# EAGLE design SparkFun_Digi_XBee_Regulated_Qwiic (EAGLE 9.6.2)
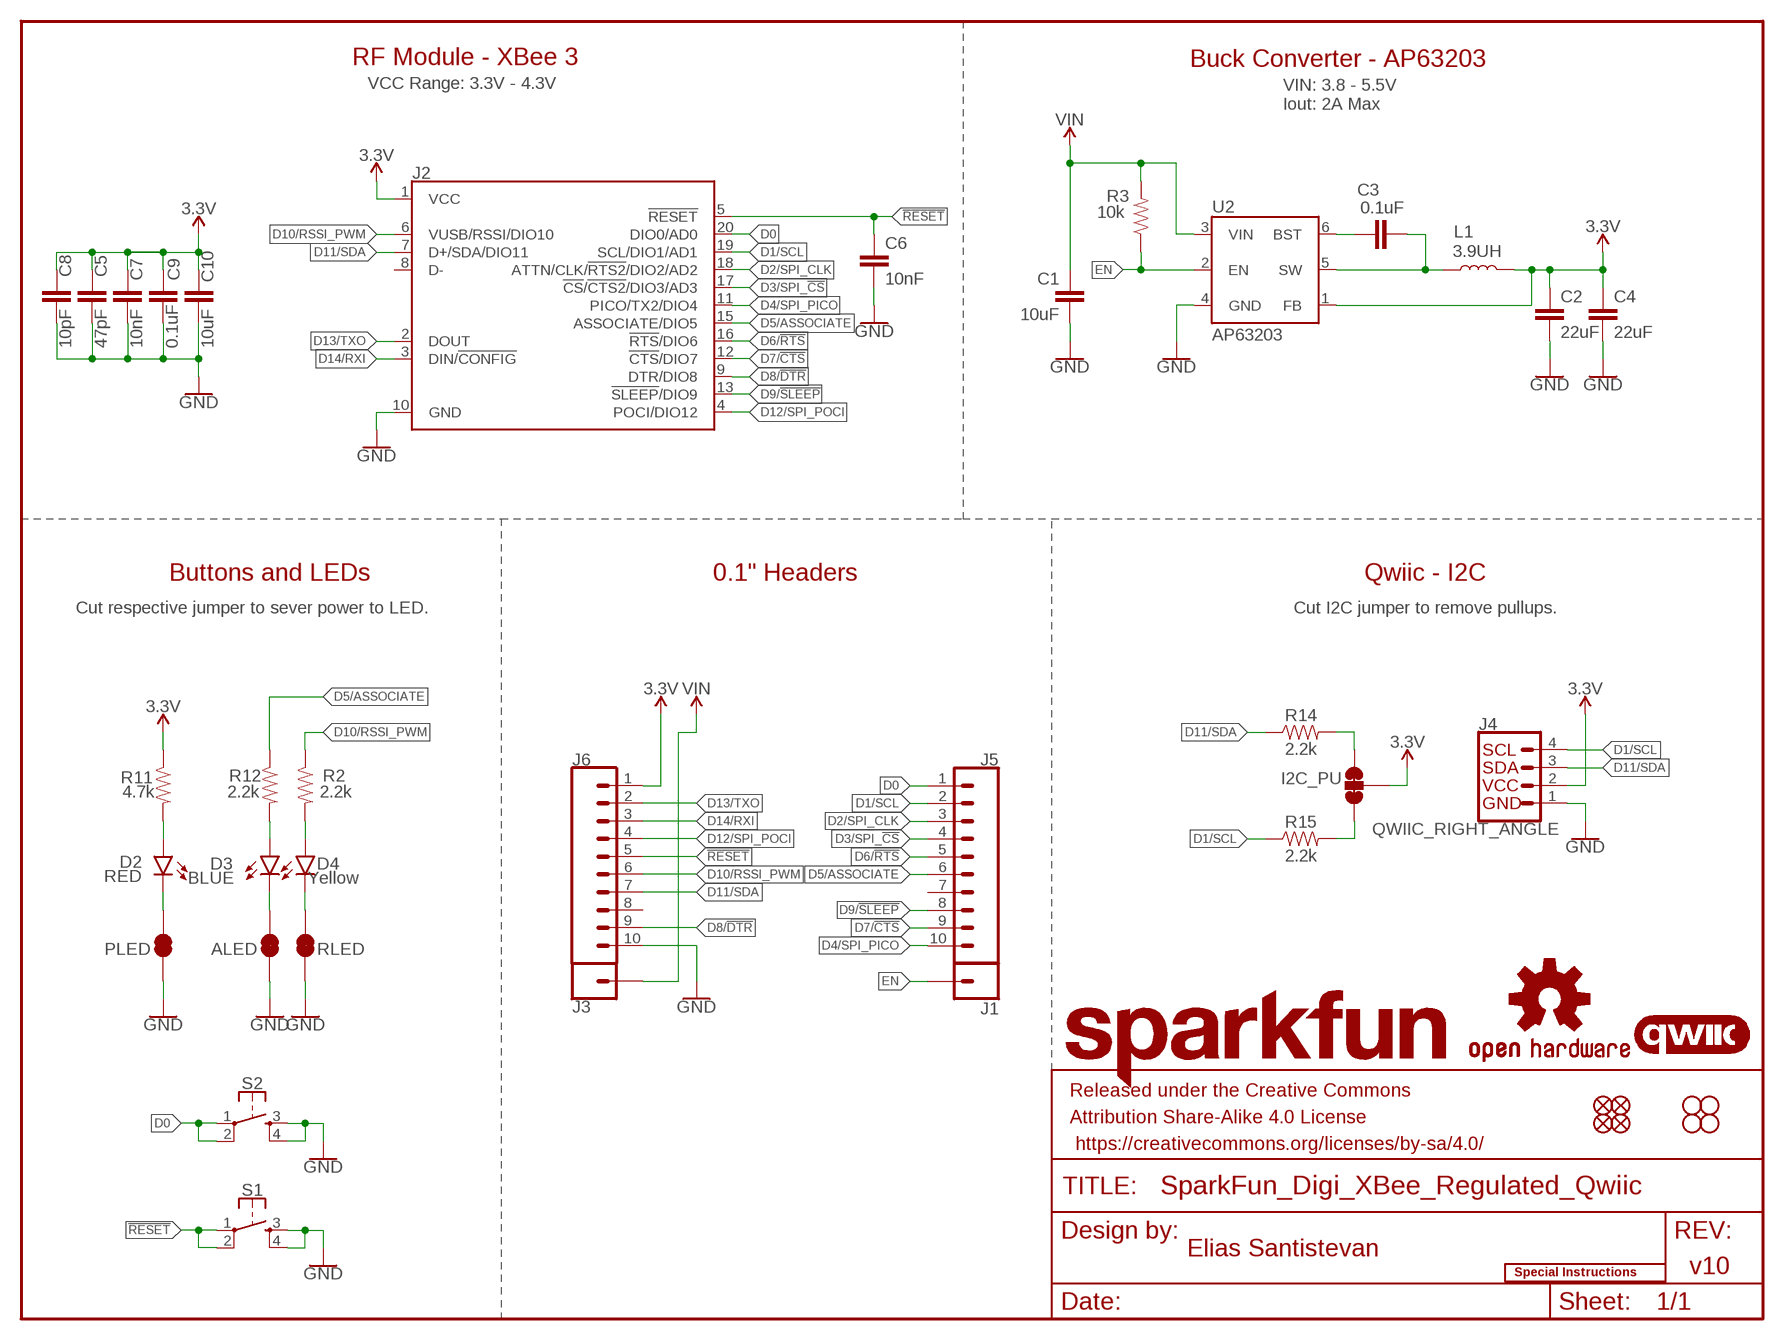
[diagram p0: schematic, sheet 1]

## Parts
ALED  JUMPER-SMT_2_NC_TRACE_SILK  [SMT-JUMPER_2_NC_TRACE_SILK]
C1  10uF  10UF-1210-50V-20%  [1210]
C2  22uF  22UF-0603-6.3V-20%  [0603]
C3  0.1uF  0.1UF-0603-25V-5%  [0603]
C4  22uF  22UF-0603-6.3V-20%  [0603]
C5  47pF  47PF-0603-50V-5%  [0603]
C6  10nF  10NF-0603-50V-10%  [0603]
C7  10nF  10NF-0603-50V-10%  [0603]
C8  10pF  10PF-0603-50V-5%  [0603]
C9  0.1uF  0.1UF-0603-25V-(+80/-20%)  [0603]
C10  10uF  10UF-0603-6.3V-20%  [0603]
D2  RED  LED-RED_0603-KB  [LED-0603]
D3  BLUE  LED-BLUE0603  [LED-0603]
D4  Yellow  LED-YELLOW0603  [LED-0603]
FD1  FIDUCIAL1X2  [FIDUCIAL-1X2]
FD2  FIDUCIAL1X2  [FIDUCIAL-1X2]
FD3  FIDUCIAL1X2  [FIDUCIAL-1X2]
FD4  FIDUCIAL1X2  [FIDUCIAL-1X2]
FRAME2  FRAME-LETTER  [CREATIVE_COMMONS]
H1  STAND-OFFTIGHT  [STAND-OFF-TIGHT]
H2  STAND-OFFTIGHT  [STAND-OFF-TIGHT]
H3  STAND-OFFTIGHT  [STAND-OFF-TIGHT]
H4  STAND-OFFTIGHT  [STAND-OFF-TIGHT]
I2C_PU  JUMPER-SMT_3_2-NC_TRACE_SILK  [SMT-JUMPER_3_2-NC_TRACE_SILK]
J1  CONN_01PTH_NO_SILK_STAND  [1X01_NO_SILK_STAND]
J2  XBEE_UPDATEXBEE_SMD  [XBEE3-SMD]
J3  CONN_01PTH_NO_SILK_STAND  [1X01_NO_SILK_STAND]
J4  QWIIC_RIGHT_ANGLE  QWIIC_CONNECTORJS-1MM  [JST04_1MM_RA]
J5  CONN_10NO_SILK_PTH_FEMALE  [1X10_NO_SILK]
J6  CONN_10NO_SILK_PTH_FEMALE  [1X10_NO_SILK]
L1  3.9UH  [INDUCTOR_3.9UH]
LOGO1  SPECIAL_INSTRUCTIONS-ORDERING  [ORDERING_INSTRUCTIONS]
LOGO2  OSHW-LOGOS  [OSHW-LOGO-S]
LOGO3  QWIIC_LOGO_4MM  [QWIIC_4MM]
LOGO4  SFE_LOGO_NAMEBLANK  [BLANK]
PLED  JUMPER-SMT_2_NC_TRACE_SILK  [SMT-JUMPER_2_NC_TRACE_SILK]
R2  2.2k  2.2KOHM-0603-1/10W-1%  [0603]
R3  10k  10KOHM-0603-1/10W-1%  [0603]
R11  4.7k  4.7KOHM-0603-1/10W-1%  [0603]
R12  2.2k  2.2KOHM-0603-1/10W-1%  [0603]
R14  2.2k  2.2KOHM-0603-1/10W-1%  [0603]
R15  2.2k  2.2KOHM-0603-1/10W-1%  [0603]
RLED  JUMPER-SMT_2_NC_TRACE_SILK  [SMT-JUMPER_2_NC_TRACE_SILK]
S1  MOMENTARY-SWITCH-SPST-2-SMD-5.2MM-TALL  [TACTILE_SWITCH_SMD_5.2MM]
S2  MOMENTARY-SWITCH-SPST-2-SMD-5.2MM-TALL  [TACTILE_SWITCH_SMD_5.2MM]
U2  AP63203  [SOT23-6]

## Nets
3.3V: C2.1 C4.1 C5.1 C7.1 C8.1 C9.1 C10.1 I2C_PU.2 J2.1(VCC) J4.2 J6.1 L1.P$2 R11.1 U2.1(FB)
!RESET!: C6.1 J2.5(!RESET!) J6.5 S1.1 S1.2
D0: J2.20(DIO0/AD0) J5.1 S2.1 S2.2
D1/SCL: J2.19(SCL/DIO1/AD1) J4.4 J5.2 R15.1
D2/SPI_CLK: J2.18(ATTN/CLK/!RTS2!/DIO2/AD2) J5.3
D3/SPI_!CS!: J2.17(!CS!/!CTS2!/DIO3/AD3) J5.4
D4/SPI_PICO: J2.11(PICO/TX2/DIO4) J5.10
D5/ASSOCIATE: J2.15(ASSOCIATE/DIO5) J5.6 R12.1
D6/!RTS!: J2.16(!RTS!/DIO6) J5.5
D7/!CTS!: J2.12(!CTS!/DIO7) J5.9
D8/!DTR!: J2.9(DTR/DIO8) J6.9
D9/!SLEEP!: J2.13(!SLEEP!/DIO9) J5.8
D10/RSSI_PWM: J2.6(VUSB/RSSI/DIO10) J6.6 R2.1
D11/SDA: J2.7(D+/SDA/DIO11) J4.3 J6.7 R14.1
D12/SPI_POCI: J2.4(POCI/DIO12) J6.4
D13/TXO: J2.2(DOUT) J6.2
D14/RXI: J2.3(DIN/!CONFIG!) J6.3
EN: J1.1 R3.1 U2.2(EN)
GND: ALED.1 C1.2 C2.2 C4.2 C5.2 C6.2 C7.2 C8.2 C9.2 C10.2 J2.10(GND) J4.1 J6.10 PLED.1 RLED.1 S1.3 S1.4 S2.3 S2.4 U2.4(GND)
N$1: C3.1 U2.6(BST)
N$2: D4.A R2.2
N$3: D4.C RLED.2
N$7: D2.A R11.2
N$8: C3.2 L1.P$1 U2.5(SW)
N$11: I2C_PU.3 R14.2
N$12: D3.A R12.2
N$13: I2C_PU.1 R15.2
N$21: ALED.2 D3.C
N$23: D2.C PLED.2
VIN: C1.1 J3.1 R3.2 U2.3(VIN)
Unconnected: J2.8(D-) J5.7 J6.8

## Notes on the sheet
- RF Module - XBee 3 | Buck Converter - AP63203
- VCC Range: 3.3V - 4.3V
- VIN: 3.8 - 5.5V
  Iout: 2A Max
- Buttons and LEDs | 0.1" Headers | Qwiic - I2C
- Cut respective jumper to sever power to LED. | Cut I2C jumper to remove pullups.
- Elias Santistevan
- v10

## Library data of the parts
ALED PLED RLED = SparkFun-Jumpers:JUMPER-SMT_2_NC_TRACE: Normally closed trace jumper
C1 = SparkFun-Capacitors:10UF: 10.0µF ceramic capacitors; PROD_ID: CAP-09824
C2 C4 = SparkFun-Capacitors:22UF: 22µF ceramic capacitors; PROD_ID: CAP-14464
C3 = SparkFun-Capacitors:0.1UF: 0.1µF ceramic capacitors; PROD_ID: CAP-08604
C5 = SparkFun-Capacitors:47PF: 47pF ceramic capacitors; PROD_ID: CAP-08913
C6 C7 = SparkFun-Capacitors:10NF: 0.01uF/10nF/10,000pF ceramic capacitors; PROD_ID: CAP-00867
C8 = SparkFun-Capacitors:10PF: 10pF ceramic capacitors; PROD_ID: CAP-11812
C9 = SparkFun-Capacitors:0.1UF: 0.1µF ceramic capacitors; PROD_ID: CAP-00810
C10 = SparkFun-Capacitors:10UF: 10.0µF ceramic capacitors; PROD_ID: CAP-11015
D2 = SparkFun-LED:LED-RED: Red SMD LED; PROD_ID: DIO-17976
D3 = SparkFun-LED:LED-BLUE: Blue SMD LED; PROD_ID: DIO-08575
D4 = SparkFun-LED:LED-YELLOW: Yellow SMD LED; PROD_ID: DIO-09003
FD1-FD4 = SparkFun-Aesthetics:FIDUCIAL: Fiducial Alignment Points
FRAME2 = SparkFun-Aesthetics:FRAME-LETTER: Schematic Frame - Letter
H1-H4 = SparkFun-Hardware:STAND-OFF: Stand Off
I2C_PU = SparkFun-Jumpers:JUMPER-SMT_3_2-NC_TRACE: Normally closed trace jumper (2 of 2 connections) This jumper has a trace between all three pads so they are normally closed (NC). Use a razor knife to open the connection(s). For best results follow the IPC guidelines for cutting traces: Cutout at least 0.063 mm (0.005 in). Remove all loose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
J1 J3 = SparkFun-Connectors:CONN_01: Single connection point. Often used as Generic Header-pin footprint for 0.1 inch spaced/style header connections
J2 = xbee_smart_modem:XBEE_UPDATE: XBee 3 Cat 1 Smart Modem
J4 = SparkFun-Connectors:QWIIC_CONNECTOR: SparkFun I2C Standard Qwiic Connector An SMD 1mm pitch JST connector makes it easy and quick (get it? Qwiic?) to connect I2C devices to each other. The Qwiic system enables fast and solderless connection between popular platforms and various sensors and actuators. We carry 200mm, 100mm, 50mm, and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; PROD_ID: CONN-13694
J5 J6 = SparkFun-Connectors:CONN_10: Multi connection point. Often used as Generic Header-pin footprint for 0.1 inch spaced/style header connections On any of the 0.1 inch spaced packages, you can populate with these: Break Away Headers - Straight (PRT-00116) Break Away Male Headers - Right Angle (PRT-00553) Female Headers (PRT-00115)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
L1 = SparkFun-Coils:3.9UH: Würth's Electronik 3.9uH Inductor; PROD_ID: NDUC-18014
LOGO1 = SparkFun-Aesthetics:SPECIAL_INSTRUCTIONS: Special Ordering/Production Instructions Alert
LOGO2 = SparkFun-Aesthetics:OSHW-LOGO: Open-Source Hardware (OSHW) Logo
LOGO3 = SparkFun-Aesthetics:QWIIC_LOGO: Qwiic Logos for placement on schematic and PCB. The 5.5mm silk logo is best for placing next to Qwiic connector.
LOGO4 = SparkFun-Aesthetics:SFE_LOGO_NAME: SparkFun Font Logo
R2 R12 R14 R15 = SparkFun-Resistors:2.2KOHM: 2.2kΩ resistor; PROD_ID: RES-08272
R3 = SparkFun-Resistors:10KOHM: 10kΩ resistor; PROD_ID: RES-00824
R11 = SparkFun-Resistors:4.7KOHM: 4.7kΩ resistor; PROD_ID: RES-07857
S1 S2 = SparkFun-Switches:MOMENTARY-SWITCH-SPST-2: Momentary Switch (Pushbutton) - SPST - Two Circuits Normally-open (NO) SPST momentary switches (buttons, pushbuttons). Schematic symbol includes two switch circuits. Variants SMD-4.6MMX2.8MM - 4.60mm x 2.80mm Tactile Momentary Button Switch - Used on SparkFun Pro Micro - RP2040 SMD-5.2MM - Mini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; PROD_ID: SWCH-14139
U2 = SparkFun-IC-Power:AP63203: Diodes Inc. AP63203 3.8V-32V input 3.3V Buck The AP63200/AP63201/AP63203/AP63205 is a 2A, synchronous buck converter with a wide input voltage range of 3.8V to 32V and fully integrates a 125mΩ high-side power MOSFET and a 68mΩ lowside power MOSFET to provide high-efficiency step-down DC/DC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; PROD_ID: VREG-15244

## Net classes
1 POWER: width 0.559 mm, drill 0.305 mm
2 Diff pairs: width 0.203 mm, drill 0.305 mm, clearance 0.152 mm

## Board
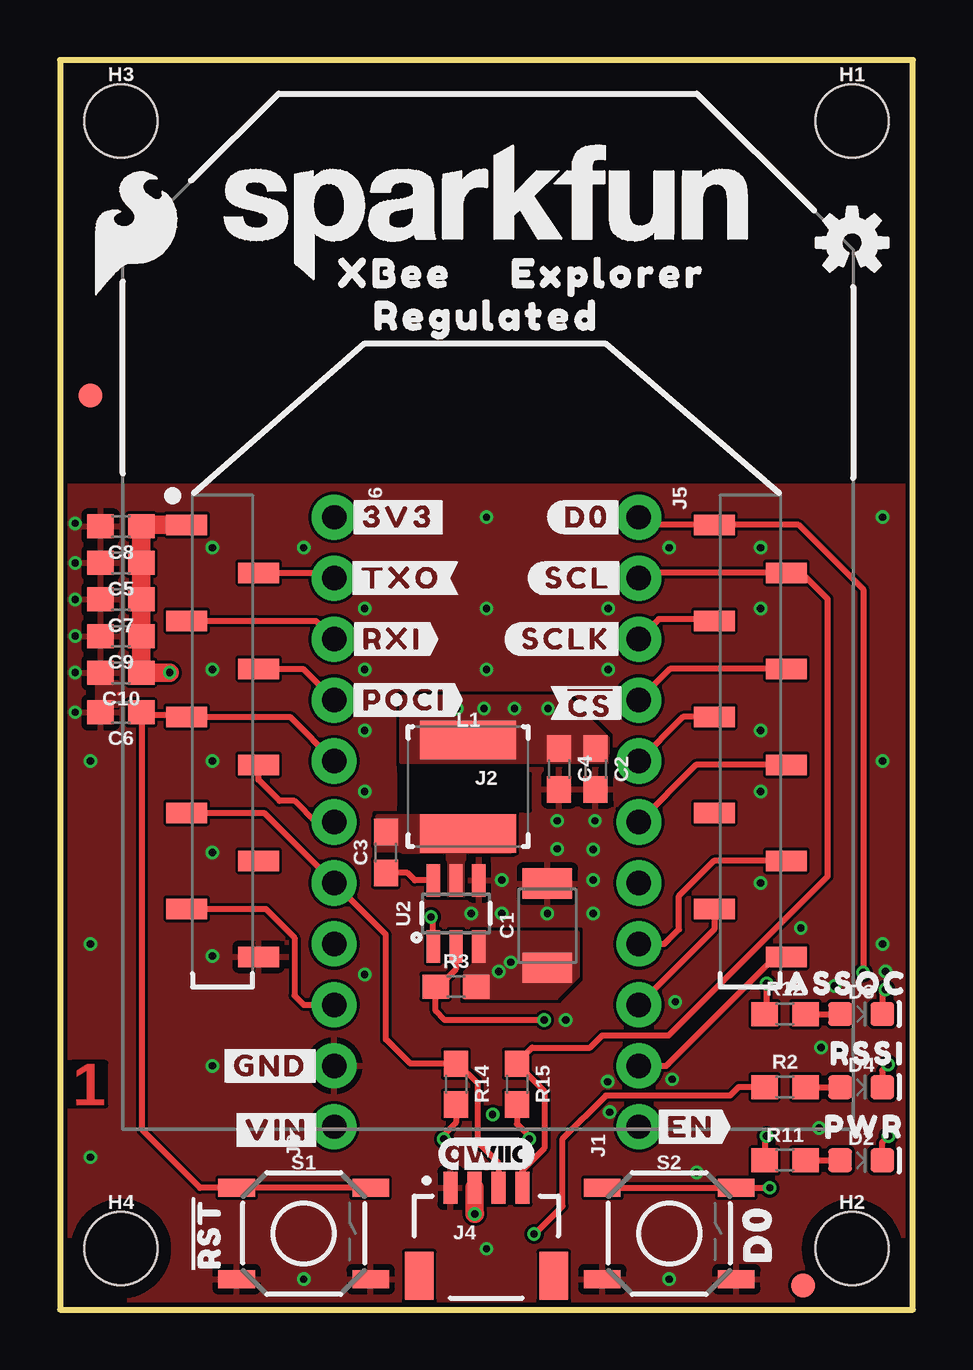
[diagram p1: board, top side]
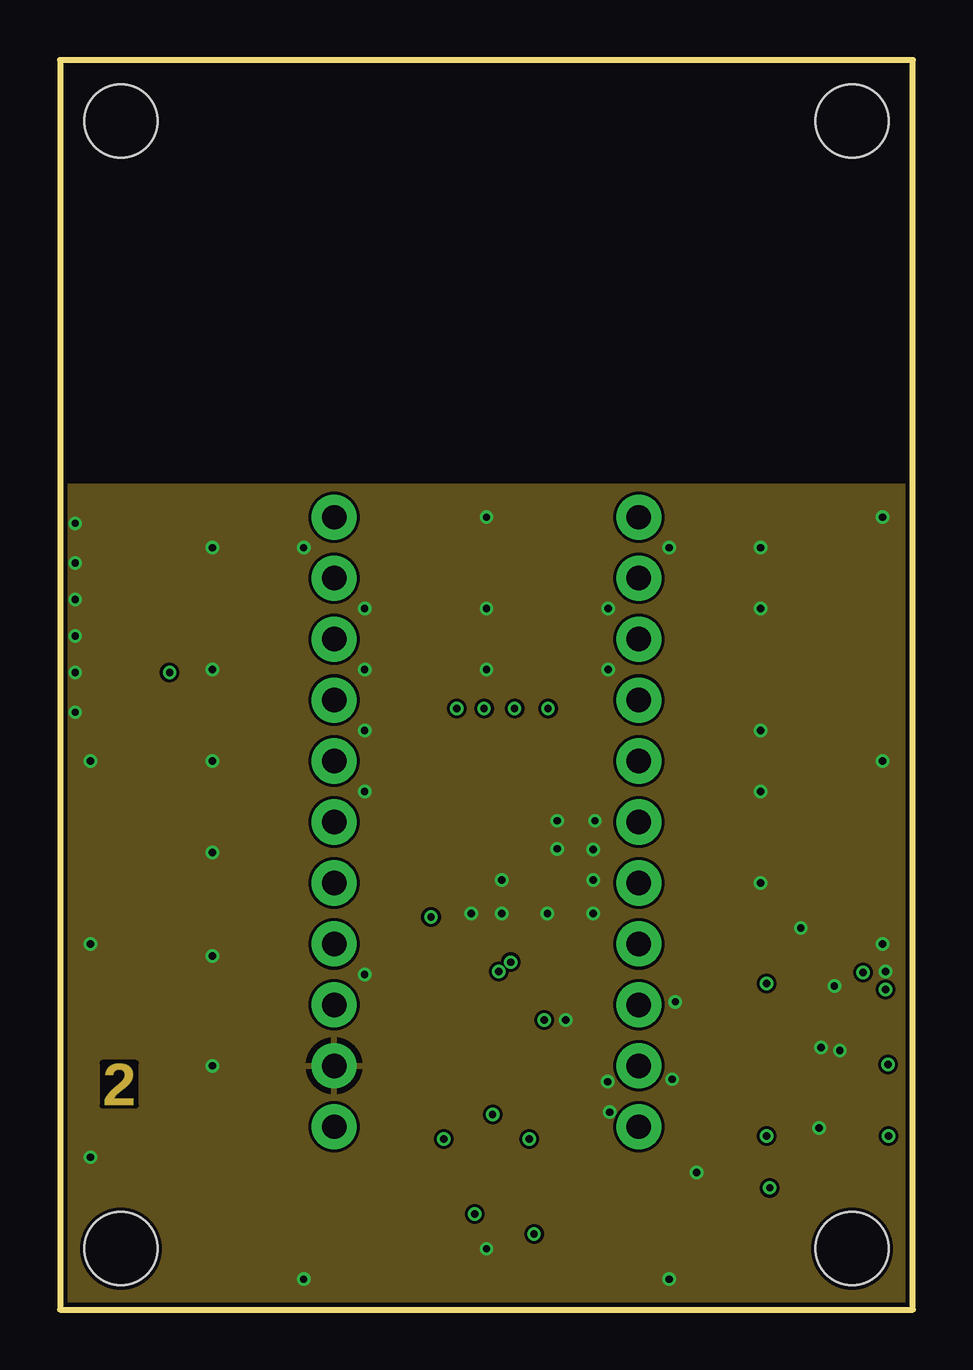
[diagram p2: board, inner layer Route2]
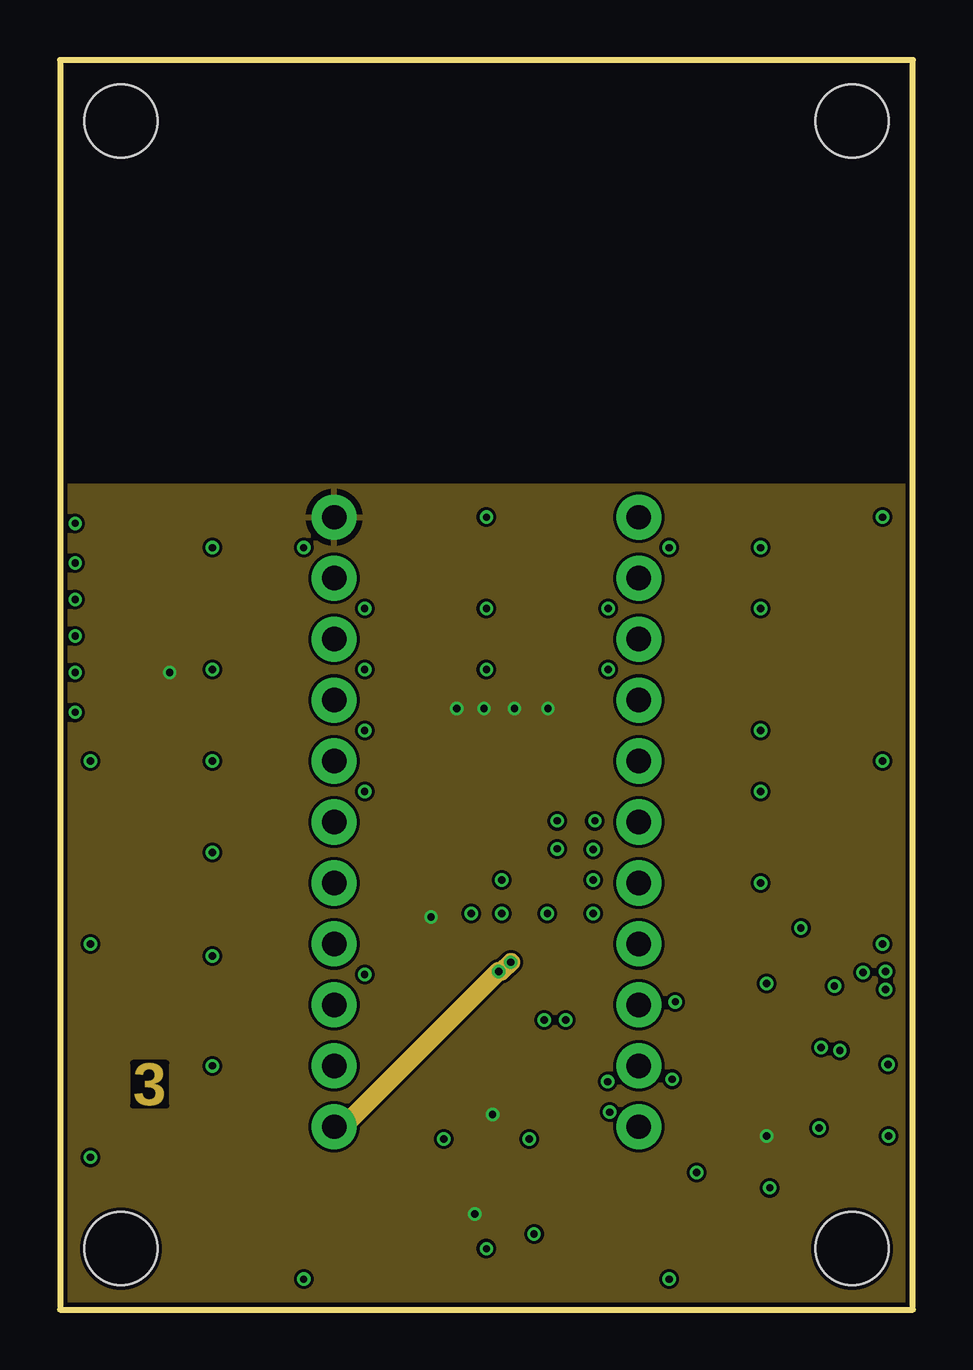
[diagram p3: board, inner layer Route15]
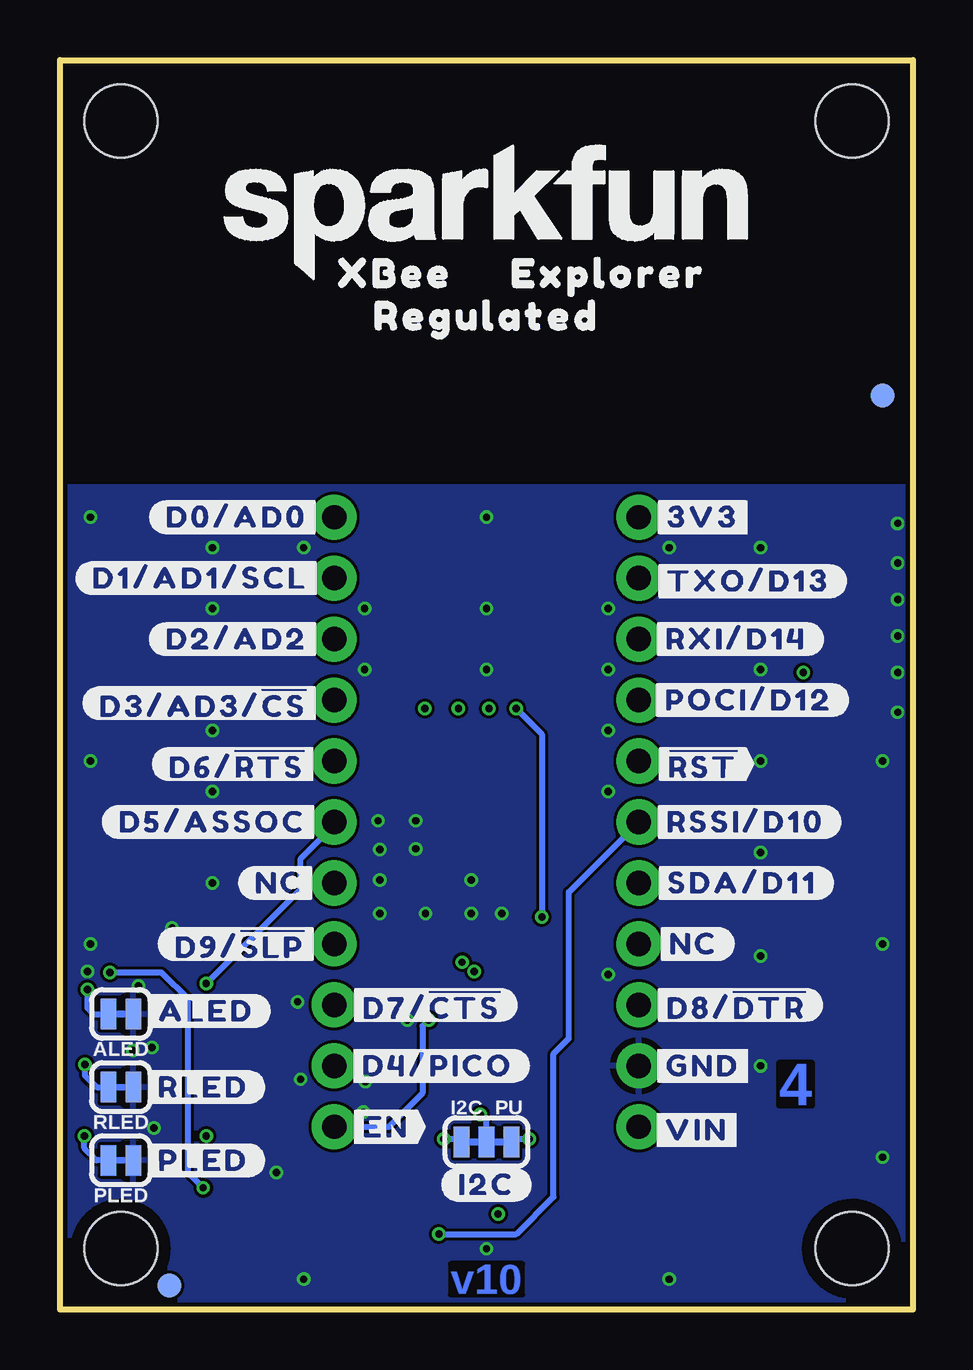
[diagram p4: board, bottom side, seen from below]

Size 35.56 x 52.07 mm. Coordinates in mm from the lower left corner, seen from the top.
Outline: 0,52.07 0,0 35.56,0 35.56,52.07 0,52.07
Copper layers (1*2*15*16): Top 0.035559375mm / dielectric 0.47751875mm / Route2 0.035559375mm / dielectric 0.47751875mm / Route15 0.035559375mm / dielectric 0.47751875mm / Bottom 0.035559375mm
Design rules "SparkFun-4-Layer-Minimum-JLCPCB": minimum track width 5mil, minimum drill 0.2mm, track to track 5mil, track to pad 5mil, pad to pad 5mil, via to via 5mil, smd to smd 5mil, copper to edge 7mil, drill to drill 7mil, minimum pad ring 5mil, minimum via ring 5mil, stop-mask expansion 2.5mil, vias tented up to drill 25mil, thermal gap 10mil
tRestrict: area 14.2,21 to 14.4,22.4; area 19.4,20.8 to 19.6,22.3

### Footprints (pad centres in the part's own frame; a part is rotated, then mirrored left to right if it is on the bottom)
SMT-JUMPER_2_NC_TRACE_SILK = smd 0.66 x 1.27: 1 -0.521,0; 2 0.521,0
1210 = smd 1.27 x 2.06: 1 -1.755,0; 2 1.755,0
0603 = smd 1.1 x 1: 1 -0.85,0; 2 0.85,0
LED-0603 = smd 1 x 1: A -0.877,0; C 0.877,0
FIDUCIAL-1X2 = smd 1 x 1: 1 0,0
STAND-OFF-TIGHT = hole 3.048: 0,0
SMT-JUMPER_3_2-NC_TRACE_SILK = smd 0.66 x 1.27: 1 -1.041,0; 2 0,0; 3 1.041,0
1X01_NO_SILK_STAND = drill 1.016 pad 1.88: 1 0,0
XBEE3-SMD = smd 1.7 x 0.85: 1 -12.5,11.11; 2 -9.5,9.11; 3 -12.5,7.11; 4 -9.5,5.11; 5 -12.5,3.11; 6 -9.5,1.11; 7 -12.5,-0.89; 8 -9.5,-2.89; 9 -12.5,-4.89; 10 -9.5,-6.89; 11 12.5,-6.89; 12 9.5,-4.89; 13 12.5,-2.89; 14 9.5,-0.89; 15 12.5,1.11; 16 9.5,3.11; 17 12.5,5.11; 18 9.5,7.11; 19 12.5,9.11; 20 9.5,11.11
JST04_1MM_RA = smd 0.6 x 1.35: 1 -1.5,0; 2 -0.5,0; 3 0.5,0; 4 1.5,0 | smd 1.2 x 2: NC1 2.8,-3.675; NC2 -2.8,-3.675
1X10_NO_SILK = drill 1.016 pad 1.88: 1 0,0; 2 2.54,0; 3 5.08,0; 4 7.62,0; 5 10.16,0; 6 12.7,0; 7 15.24,0; 8 17.78,0; 9 20.32,0; 10 22.86,0
INDUCTOR_3.9UH = smd 4 x 1.6: P$1 0,-2; P$2 0,1.9
TACTILE_SWITCH_SMD_5.2MM = smd 1.524 x 0.762: 1 -2.794,1.905; 2 2.794,1.905; 3 -2.794,-1.905; 4 2.794,-1.905
SOT23-6 = smd 0.55 x 1.35: 1 -0.95,-1.375; 2 0,-1.375; 3 0.95,-1.375; 4 0.95,1.375; 5 0,1.375; 6 -0.95,1.375

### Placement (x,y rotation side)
ALED  33.02,12.32 180 bottom
C1  20.32,16 90 top
C2  22.33,22.53 270 top
C3  13.59,19.05 90 top
C4  20.8,22.53 270 top
C5  2.54,31.11 180 top
C6  2.54,24.89 180 top
C7  2.54,29.59 180 top
C8  2.54,32.64 180 top
C9  2.54,28.07 180 top
C10  2.54,26.54 180 top
D2  33.4,6.22 0 top
D3  33.4,12.32 0 top
D4  33.4,9.27 0 top
FD1  1.27,38.1 0 top
FD2  1.27,38.1 0 bottom
FD3  30.99,1.02 0 top
FD4  30.99,1.02 0 bottom
FRAME2  not placed on the board
H1  33.02,49.53 0 top
H2  33.02,2.54 0 top
H3  2.54,49.53 0 top
H4  2.54,2.54 0 top
I2C_PU  17.78,6.99 0 bottom
J1  24.13,7.62 90 top
J2  17.78,21.59 0 top
J3  11.43,7.62 90 top
J4  17.78,5.08 0 top
J5  24.13,33.02 270 top
J6  11.43,33.02 270 top
L1  17.02,21.84 0 top
LOGO1  not placed on the board
LOGO2  33.02,44.45 0 top
LOGO3  17.78,6.48 0 top
LOGO4  not placed on the board
PLED  33.02,6.22 180 bottom
R2  30.23,9.27 0 top
R3  16.51,13.46 0 top
R11  30.23,6.22 0 top
R12  30.23,12.32 0 top
R14  16.51,9.4 270 top
R15  19.05,9.4 270 top
RLED  33.02,9.27 180 bottom
S1  10.16,3.17 0 top
S2  25.4,3.17 0 top
U2  16.51,16.51 0 top
U$1  [#GND#0]  8.76,10.16 0 top
U$2  [SFE_LOGO_NAME_.2]  17.78,45.72 0 top
U$3  [#EN#17]  21.97,7.62 0 bottom
U$4  [#NC#1]  9.14,15.24 0 bottom
U$5  [#NC#3]  26.42,17.78 0 bottom
U$6  [#EN#17]  26.29,7.62 0 top
U$7  [#D7##CTS##26]  20.07,12.7 0 bottom
U$8  [#D0#AD0#18]  28.19,33.02 0 bottom
U$9  [#3V3#1]  14.1,33.02 0 top
U$10  [#D4#PICO#25]  19.81,10.16 0 bottom
U$11  [#RLED#22]  29.59,9.27 0 bottom
U$12  [#GND#0]  8.76,10.16 0 bottom
U$13  [#D8##DTR##27]  7.37,12.7 0 bottom
U$14  [#RSSI#D10#17]  6.98,20.32 0 bottom
U$15  [#SDA#D11#9]  7.11,17.78 0 bottom
U$16  [##RST##15]  8.76,22.73 0 bottom
U$17  [#POCI#D12#24]  6.86,25.4 0 bottom
U$18  [#RXI#D14#15]  7.37,27.94 0 bottom
U$19  [#D2#AD2#19]  28.19,27.94 0 bottom
U$20  [#D6##RTS##25]  28.19,22.73 0 bottom
U$21  [#TXO#8]  14.22,30.48 0 top
U$22  [#TXO#D13#13]  6.86,30.35 0 bottom
U$23  [EXPLORER1344]  12.7,43.18 0 bottom
U$24  [REGULATED1343]  17.78,41.4 0 bottom
U$25  [XBEE340]  21.59,43.18 0 bottom
U$26  [#I2C#33]  17.78,5.21 0 bottom
U$27  [#RXI#7]  13.84,27.94 0 top
U$28  [XBEE340]  13.97,43.18 0 top
U$29  [REGULATED1343]  17.78,41.4 0 top
U$30  [#RST#30]  6.1,3.17 90 top
U$31  [#D0#3]  21.97,33.02 0 top
U$32  [#D1#AD1#SCL#8]  29.72,30.48 0 bottom
U$33  [EXPLORER1344]  22.86,43.18 0 top
U$34  [#D3#AD3##CS##23]  29.59,25.27 0 bottom
U$35  [#D5#ASSOC#25]  29.21,20.32 0 bottom
U$36  [#D9##SLP##28]  28.07,15.24 0 bottom
U$40  [D03]  29.08,3.17 90 top
U$42  [PWR26]  33.53,7.62 0 top
U$43  [ASSOC27]  32.77,13.59 0 top
U$44  [#3V3#1]  8.76,33.02 0 bottom
U$45  [#POCI#32]  14.35,25.4 0 top
U$46  [#VIN#4]  9.02,7.49 0 bottom
U$49  [#ALED#21]  29.46,12.45 0 bottom
U$52  [#PLED#20]  29.59,6.22 0 bottom
U$59  [##CS##26]  22.1,25.27 0 top
U$60  [#SCLK#33]  21.08,27.94 0 top
U$61  [SFE_LOGO_FLAME_.2]  3.17,44.83 0 top
U$62  [RSSI31]  33.66,10.67 0 top
U$63  [SFE_LOGO_NAME_.2]  17.78,45.72 0 bottom
U$64  [#SCL#9]  21.59,30.48 0 top
U$65  [#D0#3]  21.97,33.02 0 top
U$66  [#VIN#4]  9.02,7.49 0 top

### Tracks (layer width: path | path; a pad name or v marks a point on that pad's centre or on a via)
3.3V  (via drill 0.3)
  Top 0.254: v29.46,7.24 29.38,7.15 R11.1 | v15.47,16.36 15.56,16.27 U2.1
  Top 0.762: J4.2 17.28,4 v17.3,3.99 | J2.1 3.45,32.7 C8.1 C5.1 C7.1 C9.1 C10.1 v4.57,26.54
  Bottom 0.254: v16.54,25.04 15.47,23.98 v15.47,16.36 | I2C_PU.2 17.78,7.87 v18.03,8.13
  other vias: 17.68,25.04 18.95,25.04 20.35,25.04
  pour Top (isolate 0.305, no thermals): 22.83,22.78 14.22,22.78 14.22,25.58 21.11,25.58 22.83,23.85
  pour Route15 (isolate 0.127, rank 3): 0,0 35.56,0 35.56,34.29 0,34.29
!RESET!
  Top 0.254: J6.5 9.59,24.7 J2.5 5.21,24.77 3.52,24.77 C6.1 3.43,24.85 3.43,7.49 5.84,5.08 S1.1 S1.2
D0  (via drill 0.3)
  Top 0.254: J5.1 24.45,32.7 J2.20 30.8,32.7 33.48,30.02 v33.48,14.05 | S2.1 S2.2 v29.59,5.08
  Bottom 0.254: v29.59,5.08 30.23,5.71 30.23,12.95 31.32,14.05 v33.48,14.05
D1/SCL
  Top 0.254: J5.2 24.35,30.7 J2.19 30.91,30.7 32,29.61 32,18.06 25.38,11.43 22.61,11.43 22.1,10.92 19.68,10.92 19.05,10.29 R15.1 20.19,9.11 20.19,6.73 19.28,5.82 J4.4
D2/SPI_CLK
  Top 0.254: J2.18 27.2,28.78 24.97,28.78 J5.3
D3/SPI_!CS!
  Top 0.254: J5.4 25.43,26.7 J2.17
D4/SPI_PICO
  Top 0.254: J5.10 25.27,10.16 29.81,14.7 J2.11
D5/ASSOCIATE  (via drill 0.3)
  Top 0.254: J2.15 26.51,22.7 J5.6 | R12.1 29.46,12.41 v29.46,13.59
  Bottom 0.254: J5.6 24.07,20.26 25.53,18.8 25.53,17.53 v29.46,13.59
D6/!RTS!
  Top 0.254: J5.5 25.97,24.7 J2.16
D7/!CTS!
  Top 0.254: J2.12 27.28,15.85 J5.9
D8/!DTR!
  Top 0.254: J2.9 8.57,16.7 9.78,15.49 9.78,13.08 10.16,12.7 J6.9
D9/!SLEEP!
  Top 0.254: J2.13 27.26,18.7 25.81,17.25 25.81,15.85 25.2,15.24 J5.8
D10/RSSI_PWM  (via drill 0.3)
  Top 0.254: J6.6 10.66,20.32 9.78,21.2 9.15,21.2 8.28,22.07 J2.6 | R2.1 28.28,9.27 27.93,8.91 22.76,8.91 20.95,7.11 20.95,4.32 19.79,3.15 v19.76,3.15
  Bottom 0.254: v19.76,3.15 16.54,3.15 14.99,4.7 14.99,10.67 14.35,11.3 14.35,17.4 J6.6
D11/SDA
  Top 0.254: J2.7 8.51,20.7 J6.7 13.59,15.62 13.59,11.26 14.61,10.25 R14.1 16.6,10.25 17.4,9.45 17.4,6.99 18.28,6.11 J4.3
D12/SPI_POCI
  Top 0.254: J2.4 10.13,26.7 J6.4
D13/TXO
  Top 0.254: J2.2 11.21,30.7 J6.2
D14/RXI
  Top 0.254: J6.3 10.67,28.7 J2.3
EN  (via drill 0.3)
  Top 0.254: U2.2 16.51,14.19 15.79,13.46 R3.1 15.66,12.45 16.04,12.06 v20.19,12.06
  Bottom 0.254: J1.1 21.84,7.62 20.45,9.02 20.45,11.81 v20.19,12.06
GND  (via drill 0.3)
  Top 0.152: 2.54,25.65 2.45,25.65
  other vias: 20.73,19.2 22.22,19.18 18.41,16.51 6.35,14.73 25.65,12.83 1.27,6.35 10.16,1.27 17.78,2.54 25.4,1.27 0.64,26.54 0.64,28.07 0.64,32.77 0.64,29.59 0.64,31.11 20.32,16.51 22.22,17.91 22.22,16.51 26.54,5.71 22.91,8.23 18.41,17.91 0.64,24.89 34.29,33.02 34.29,22.86 30.89,15.9 34.29,15.24 1.27,15.24 1.27,22.86 21.08,12.06 31.72,10.92 34.42,14.1 32.51,10.79 32.28,13.49 17.78,33.02 31.65,7.57 22.83,9.5 6.35,31.75 6.35,26.67 6.35,19.05 6.35,22.86 29.21,31.75 29.21,29.21 29.21,24.13 29.21,21.59 29.21,17.78 25.4,31.75 10.16,31.75 17.78,29.21 17.78,26.67 22.86,29.21 22.86,26.67 12.7,29.21 12.7,26.67 12.7,21.59 12.7,13.97 6.35,10.16 25.53,9.6 22.3,20.37 20.73,20.37 12.7,24.13 17.14,16.51
  pour Top (isolate 0.127, rank 3): 0,0 35.56,0 35.56,34.29 0,34.29
  pour Bottom (isolate 0.127, rank 3): 0,0 35.56,0 35.56,34.29 0,34.29
  pour Route2 (isolate 0.127, rank 3): 0,0 35.56,0 35.56,34.29 0,34.29
  pour Top (isolate 0.305, no thermals): 1.52,26.16 2.41,26.16 2.92,25.65 2.41,25.15 1.52,25.15
N$1
  Top 0.254: U2.6 14.8,17.89 14.48,18.2 C3.1
N$2
  Top 0.254: R2.2 D4.A
N$3  (via drill 0.3)
  Top 0.254: v34.52,10.21 34.28,9.97 D4.C
  Bottom 0.254: v34.52,10.21 34.52,9.75 34.04,9.27 RLED.2
N$7
  Top 0.254: R11.2 D2.A
N$8
  pour Top (isolate 0.305, no thermals): 16.89,17.27 16.89,19.05 18.8,19.05 18.8,20.57 13.21,20.57 13.21,19.05 16.13,19.05 16.13,17.27
N$11  (via drill 0.3)
  Top 0.254: R14.2 16.51,7.79 16,7.28 v16,7.11
  Bottom 0.254: I2C_PU.3 16.61,7.11 v16,7.11
N$12
  Top 0.254: R12.2 D3.A
N$13  (via drill 0.3)
  Top 0.254: R15.2 19.05,7.75 19.56,7.24 v19.56,7.11
  Bottom 0.254: v19.56,7.11 18.95,7.11 I2C_PU.1
N$21  (via drill 0.3)
  Top 0.254: v34.42,13.34 34.28,13.2 D3.C
  Bottom 0.254: v34.42,13.34 34.42,12.57 34.16,12.32 ALED.2
N$23  (via drill 0.3)
  Top 0.254: D2.C 34.28,6.97 v34.54,7.24
  Bottom 0.254: PLED.2 34.04,6.22 34.54,6.73 v34.54,7.24
VIN  (via drill 0.3)
  Route15 0.762: J3.1 11.81,7.62 v18.29,14.1 18.41,14.1 v18.8,14.48
  pour Top (no thermals): 16.89,12.95 16.89,14.1 17.27,14.48 17.27,15.75 21.59,15.75 21.59,13.84 20.7,12.95

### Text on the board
Top: 1
Route2: 2
Route15: 3
Bottom: 4 | v10
Measures: Units in Inches
tDocu: Four Layer Board | 1.6mm Thickness | Lead Free HASL | Elias Santistevan

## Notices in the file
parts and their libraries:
SparkFun-Capacitors: Licensing: Creative Commons ShareAlike 4.0 International - https://creativecommons.org/licenses/by-sa/4.0
SparkFun-Aesthetics: Released under the Creative Commons Attribution Share-Alike 4.0 License
SparkFun-Aesthetics: https://creativecommons.org/licenses/by-sa/4.0
